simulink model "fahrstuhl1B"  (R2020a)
settings: Solver=FixedStepDiscrete  StartTime=0.0  StopTime=Inf  FixedStep=1e-4  RelTol=1e-3  EnableMultiTasking=on

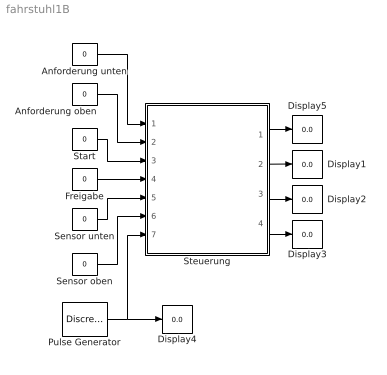
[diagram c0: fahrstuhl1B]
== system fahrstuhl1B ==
  Anforderung oben : Constant  Value=0
  Anforderung unten : Constant  Value=0
  Display{1..5} (5 alike) : Display
  Freigabe : Constant  Value=0
  Pulse Generator : DiscretePulseGenerator  PulseType=Time based  PulseWidth=50
  Sensor oben : Constant  Value=0
  Sensor unten : Constant  Value=0
  Start : Constant  Value=0
  Steuerung : Subsystem
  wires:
  Steuerung/1(Mh) -> Display5/1
  Steuerung/3(T) -> Display2/1
  Pulse Generator/1 -> Steuerung/7(Takt), Display4/1
  Sensor oben/1 -> Steuerung/6(P2)
  Sensor unten/1 -> Steuerung/5(P1)
  Freigabe/1 -> Steuerung/4(F)
  Start/1 -> Steuerung/3(S)
  Anforderung oben/1 -> Steuerung/2(A2)
  Anforderung unten/1 -> Steuerung/1(A1)
  Steuerung/4(Z) -> Display3/1
  Steuerung/2(Mr) -> Display1/1

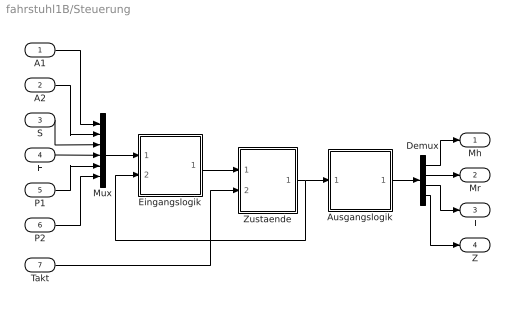
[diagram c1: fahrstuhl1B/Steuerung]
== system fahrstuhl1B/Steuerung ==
  A1 : Inport
  A2 : Inport  Port=2
  S : Inport  Port=3
  F : Inport  Port=4
  P1 : Inport  Port=5
  P2 : Inport  Port=6
  Takt : Inport  Port=7
  Ausgangslogik : Subsystem
  Demux : Demux
  Eingangslogik : Subsystem
  Mux : Mux  Inputs=6
  Zustaende : Subsystem  mask(DFlipFlop){s0=[1;0;0;0;0;0;0;0;0;0]}
      mask prompts: s0 "Initially on"
      mask help: D Flip-Flop Block
  Mh : Outport
  Mr : Outport  Port=2
  T : Outport  Port=3
  Z : Outport  Port=4
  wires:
  A1/1 -> Mux/1
  A2/1 -> Mux/2
  S/1 -> Mux/3
  F/1 -> Mux/4
  P1/1 -> Mux/5
  P2/1 -> Mux/6
  Demux/1 -> Mh/1
  Demux/2 -> Mr/1
  Demux/3 -> T/1
  Demux/4 -> Z/1
  Mux/1 -> Eingangslogik/1(E)
  Takt/1 -> Zustaende/2(CLK)
  Zustaende/1(Q) -> Ausgangslogik/1(E), Eingangslogik/2(Z)
  Ausgangslogik/1(A) -> Demux/1
  Eingangslogik/1(A) -> Zustaende/1(D)

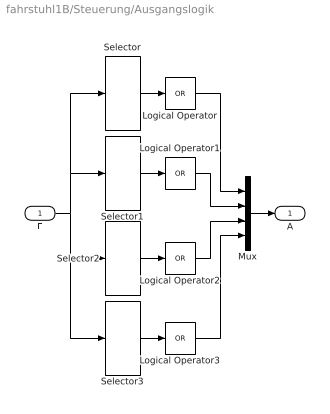
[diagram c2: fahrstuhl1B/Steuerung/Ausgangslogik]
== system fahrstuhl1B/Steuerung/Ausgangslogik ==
  E : Inport
  Logical Operator{,1..3} (4 alike) : Logic  Operator=OR  Inputs=1  AllPortsSameDT=off  OutDataTypeStr=boolean
  Mux : Mux
  Selector : Selector  InputPortWidth=10  IndexOptions=Index vector (dialog)  Indices=[3 10]  OutputSizes=1
  Selector1 : Selector  InputPortWidth=10  IndexOptions=Index vector (dialog)  Indices=[7 9]  OutputSizes=1
  Selector2 : Selector  InputPortWidth=10  IndexOptions=Index vector (dialog)  Indices=[2 4 6 8]  OutputSizes=1
  Selector3 : Selector  InputPortWidth=10  IndexOptions=Index vector (dialog)  Indices=[2 3 4 6 7 8 9 10]  OutputSizes=1
  A : Outport
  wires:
  Mux/1 -> A/1
  Logical Operator/1 -> Mux/1
  Selector/1 -> Logical Operator/1
  Selector1/1 -> Logical Operator1/1
  Logical Operator1/1 -> Mux/2
  Selector2/1 -> Logical Operator2/1
  Logical Operator2/1 -> Mux/3
  Selector3/1 -> Logical Operator3/1
  Logical Operator3/1 -> Mux/4
  E/1 -> Selector/1, Selector1/1, Selector2/1, Selector3/1

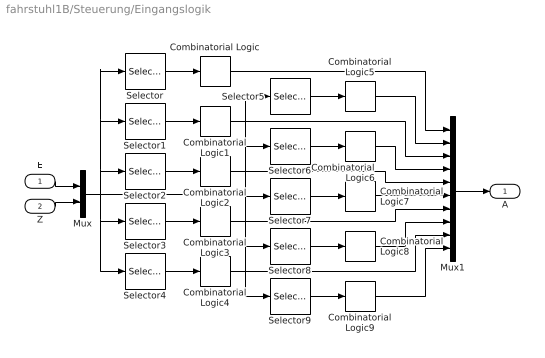
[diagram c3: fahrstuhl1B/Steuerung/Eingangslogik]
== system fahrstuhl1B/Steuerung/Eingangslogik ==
  E : Inport
  Z : Inport  Port=2
  Combinatorial Logic : CombinatorialLogic  TruthTable=[0;0;1;1;0;1;1;1;0;0;0;0;0;1;0;1;0;0;0;0;0;1;0;1;0;0;0;0;0;1;0;1]
  Combinatorial Logic{1,3..4,9} (4 alike) : CombinatorialLogic  TruthTable=[0;1;0;1;0;0;0;0;0;1;1;1;0;0;1;1]
  Combinatorial Logic2 : CombinatorialLogic  TruthTable=[0;1;0;1;0;1;1;1;0;0;0;0;0;0;1;1;0;0;0;0;0;0;1;1;0;0;0;0;0;0;1;1]
  Combinatorial Logic5 : CombinatorialLogic  TruthTable=[0;0;1;1;0;0;1;1;0;1;1;1;0;1;1;1;0;0;0;0;0;0;0;0;0;1;0;1;0;1;0;1;0;0;1;1;1;1;1;1;0;1;1;1;1;1;1;1;0;0;0;0;1;1;1;1;0;1;0;1;1;1;1;1]
  Combinatorial Logic6 : CombinatorialLogic  TruthTable=[0;1;0;1;0;1;1;1;0;0;0;0;0;0;1;1]
  Combinatorial Logic7 : CombinatorialLogic  TruthTable=[0;0;1;1;0;0;1;1;0;1;1;1;0;1;1;1;0;0;0;0;0;0;0;0;0;1;0;1;0;1;0;1;0;0;1;1;1;1;1;1;0;1;1;1;1;1;1;1;0;0;0;0;1;1;1;1;0;1;0;1;1;1;1;1]
  Combinatorial Logic8 : CombinatorialLogic  TruthTable=[0;1;0;1;0;1;1;1;0;0;0;0;0;0;1;1]
  Mux : Mux  Inputs=2
  Mux1 : Mux  Inputs=10
  Selector : Selector  InputPortWidth=16  IndexOptions=Index vector (dialog)  Indices=[1 2 4 7 14]  OutputSizes=1
  Selector1 : Selector  InputPortWidth=16  IndexOptions=Index vector (dialog)  Indices=[3 6 8 9]  OutputSizes=1
  Selector2 : Selector  InputPortWidth=16  IndexOptions=Index vector (dialog)  Indices=[1 2 4 10 11]  OutputSizes=1
  Selector3 : Selector  InputPortWidth=16  IndexOptions=Index vector (dialog)  Indices=[3 5 12 13]  OutputSizes=1
  Selector4 : Selector  InputPortWidth=16  IndexOptions=Index vector (dialog)  Indices=[1 5 11 15]  OutputSizes=1
  Selector5 : Selector  InputPortWidth=16  IndexOptions=Index vector (dialog)  Indices=[1 3 5 7 8 15]  OutputSizes=1
  Selector6 : Selector  InputPortWidth=16  IndexOptions=Index vector (dialog)  Indices=[4 6 9 10]  OutputSizes=1
  Selector7 : Selector  InputPortWidth=16  IndexOptions=Index vector (dialog)  Indices=[2 3 6 11 12 16]  OutputSizes=1
  Selector8 : Selector  InputPortWidth=16  IndexOptions=Index vector (dialog)  Indices=[4 5 13 14]  OutputSizes=1
  Selector9 : Selector  InputPortWidth=16  IndexOptions=Index vector (dialog)  Indices=[2 6 7 16]  OutputSizes=1
  A : Outport
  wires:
  Mux/1 -> Selector3/1, Selector4/1, Selector2/1, Selector1/1, Selector/1, Selector8/1, Selector9/1, Selector6/1, Selector5/1, Selector7/1
  Combinatorial Logic9/1 -> Mux1/10
  Combinatorial Logic4/1 -> Mux1/9
  Combinatorial Logic8/1 -> Mux1/8
  Combinatorial Logic3/1 -> Mux1/7
  Combinatorial Logic7/1 -> Mux1/6
  Combinatorial Logic2/1 -> Mux1/5
  Combinatorial Logic6/1 -> Mux1/4
  Combinatorial Logic1/1 -> Mux1/3
  Combinatorial Logic5/1 -> Mux1/2
  Combinatorial Logic/1 -> Mux1/1
  Mux1/1 -> A/1
  Selector9/1 -> Combinatorial Logic9/1
  Selector8/1 -> Combinatorial Logic8/1
  Selector7/1 -> Combinatorial Logic7/1
  Selector6/1 -> Combinatorial Logic6/1
  Selector5/1 -> Combinatorial Logic5/1
  Selector4/1 -> Combinatorial Logic4/1
  Selector3/1 -> Combinatorial Logic3/1
  Selector2/1 -> Combinatorial Logic2/1
  Selector1/1 -> Combinatorial Logic1/1
  Selector/1 -> Combinatorial Logic/1
  Z/1 -> Mux/2
  E/1 -> Mux/1

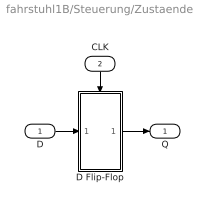
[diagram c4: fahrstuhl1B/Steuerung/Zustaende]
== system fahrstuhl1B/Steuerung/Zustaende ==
  D : Inport
  CLK : Inport  Port=2
  D Flip-Flop : Subsystem  TreatAsAtomicUnit=on
  Q : Outport  InitialOutput=0
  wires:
  D/1 -> D Flip-Flop/1(D)
  D Flip-Flop/1(Q) -> Q/1
  CLK/1 -> D Flip-Flop/Trigger

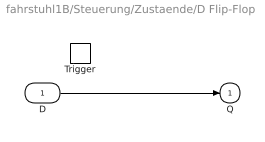
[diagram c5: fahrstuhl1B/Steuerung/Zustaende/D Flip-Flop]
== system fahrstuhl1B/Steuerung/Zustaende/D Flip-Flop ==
  D : Inport
  Trigger : TriggerPort  TriggerType=falling  VariantControl=Variant
  Q : Outport  InitialOutput=s0
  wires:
  D/1 -> Q/1
